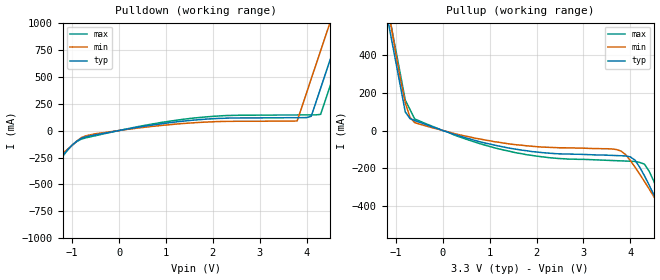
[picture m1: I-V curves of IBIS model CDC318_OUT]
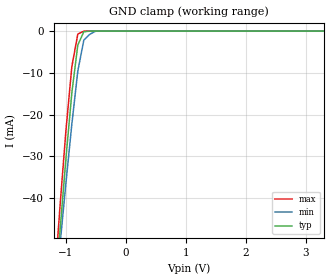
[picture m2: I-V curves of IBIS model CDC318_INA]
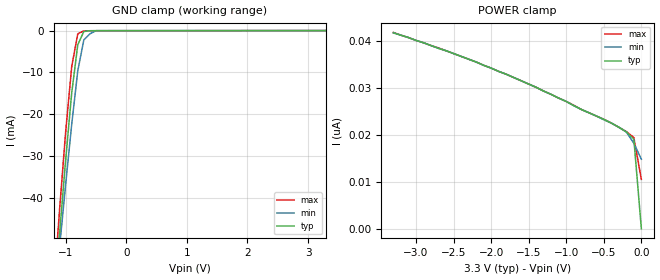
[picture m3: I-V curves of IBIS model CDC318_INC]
[IBIS Ver]   2.1
[File Name]   cd319a10.ibs
[File Rev]   1.0
[Date]   4/15/98
[Source]   file originated at Texas Instruments
[Notes]   The following information corresponds to the
|   CDC319A-DIE output buffers and input ESD circuits, derived
|   from CDC318C, the master chip of CDC319A.
|   Model names kept unchanged to show their equivalent
|   to CDC318C.
|   Only the package paracitics have been changed.
|Revision log: 1.0, 4/15/98  first revision derived from CD318C12.IBS
[Disclaimer] This information is for modeling purposes only
|and is not guaranteed.
|Property of Texas Instruments Incorporated unauthorized reproduction
|and/or distribution is strictly prohibited.
|This product is protected under copyright law and trade
|secret law as an unpublished work.  Created  1997.
|(C) Copyright 1997 Texas Instruments Incorporated.
|All rights reserved.
|These commodities are under U.S. Government distribution
|license control. As such, they are not to be re-exported
|without prior approval of the U.S. Department of Commerce.
|Please be aware that in the absence of a written agreement
|to the contrary, Texas Instruments ("TI") assumes no
|liability for:  (1) the accuracy of the IBIS Models provided
|to your company;  (2) the proper functioning of these Models
|in your design system or for any resulting applications;
|or (3) infringement of patents, copyrights or intellectual
|property rights resulting from your use of these models.
|TI provides IBIS Models as a service to our customers
|and therefore reserves the right to limit distribution
|of the Models.
|CDC319 IBIS I/O Model
|Mixed Signal Products, Texas Instruments
[Component]   CDC319   | 28-pin, DB - package
[Manufacturer] Texas Instruments
[Package]
|   typ   min   max
R_pkg   0.034   0.028   0.039
L_pkg   3.404n   2.704n   4.545n
C_pkg   0.428p   0.299p   0.571p
[Pin]  signal_name   model_name   R_pin   L_pin   C_pin
  1   VCC   POWER   0.038   4.545n   0.564p
  2   1Y0   CDC318_OUT   0.039   4.133n   0.571p
  3   1Y1   CDC318_OUT   0.035   3.598n   0.489p
  4   GND   GND   0.028   3.087n   0.408p
  5   VCC   POWER   0.032   2.990n   0.349p
  6   1Y2   CDC318_OUT   0.032   2.774n   0.318p
  7   1Y3   CDC318_OUT   0.031   2.704n   0.299p
  8   GND   GND   0.031   2.704n   0.299p
  9   A   CDC318_INA   0.032   2.774n   0.318p
 10   VCC   POWER   0.032   2.990n   0.349p
 11   3Y0   CDC318_OUT   0.028   3.087n   0.408p
 12   GND   GND   0.035   3.598n   0.489p
 13   VCC   POWER   0.039   4.133n   0.571p
 14   SDATA   CDC318_IO   0.038   4.545n   0.564p
 15   SCLOCK   CDC318_INC   0.038   4.545n   0.564p
 16   GND   GND   0.039   4.133n   0.571p
 17   GND   GND   0.035   3.597n   0.489p
 18   3Y1   CDC318_OUT   0.028   3.087n   0.408p
 19   VCC   POWER   0.032   2.990n   0.349p
 20   OE   CDC318_INE   0.031   2.774n   0.318p
 21   GND   GND   0.031   2.704n   0.299p
 22   2Y0   CDC318_OUT   0.031   2.704n   0.299p
 23   2Y1   CDC318_OUT   0.032   2.774n   0.318p
 24   VCC   POWER   0.032   2.990n   0.349p
 25   GND   GND   0.028   3.087n   0.408p
 26   2Y2   CDC318_OUT   0.035   3.598n   0.489p
 27   2Y3   CDC318_OUT   0.039   4.133n   0.571p
 28   VCC   POWER   0.038   4.545n   0.564p
| Models and submodels in the file (5): CDC318_OUT (3-state), CDC318_INA (Input), CDC318_INC (Input), CDC318_INE (Input), CDC318_IO (I/O_open_drain)
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|   Model CDC318_OUT
[Model]   CDC318_OUT
Model_type   3-state
Polarity   Non-Inverting
Enable   Active-High
Vmeas = 1.5V
Cref = 30pF
Rref = 500
Vref = 0
|   variable   typ   min   max
C_comp   5.2pF   NA   NA
[Voltage range]   3.3   3.135   3.465
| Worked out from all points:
|   slope of the pulldown table from 0 to 0.495 V, typ, clamps not added: 13.5 ohm
|   slope of the pullup table from 0 to 0.495 V, typ, clamps not added: 12.8 ohm
[Pullup]
| Voltage   I(typ)   I(min)   I(max)
-3.3V     3.358A     3.431A     3.418A
-1.2V     619mA      691mA      682mA
-1.1V     489mA      548mA      551mA
-800mV    98mA       146mA      160mA
-600mV    53mA       42mA       61mA
1.5V      -96mA      -73mA      -114mA
3.8V      -133mA     -108mA     -160mA
4.1V      -156mA     -193mA     -163mA
4.3V      -238mA     -268mA     -177mA
4.9V      -554mA     -514mA     -527mA
5V        -608mA     -556mA     -597mA
6.6V      -1.483A    -1.229A    -1.711A
[Pulldown]
|  Voltage   I(typ)   I(min)   I(max)
-3.3V     -1.354A    -1.086A    -1.669A
-2.6V     -975mA     -790mA     -1.192A
-2.3V     -813mA     -664mA     -989mA
-800mV    -71mA      -65mA      -79mA
1.6V      97mA       72mA       116mA
3.8V      119mA      89mA       144mA
4.1V      132mA      480mA      145mA
4.3V      392mA      740mA      150mA
4.5V      652mA      1A         409mA
4.7V      912mA      1.261A     669mA
4.9V      1.172A     1.521A     929mA
6.6V      3.384A     3.734A     3.137A
[Ramp]
|  variable   typ   min   max
dV/dt_r   2.00/0.95n   2.00/1.05n   2.00/0.85n
dV/dt_f   2.00/1.05n   2.00/1.15n   2.00/0.95n
|   Model CDC318_INA
[Model]   CDC318_INA
Model_type   Input
Polarity   Non-Inverting
Vinl = 0.8V
Vinh = 2.0V
Vmeas = 1.5V
| variable   typ   min   max
C_comp   3.2p   NA   NA
[Voltage range]   3.3   3.135   3.465
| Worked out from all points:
|   GND clamp passes 1 mA (typ) near -0.73 V on its own axis
[GND_Clamp]
|  Voltage   I(typ)   I(min)   I(max)
-3.3V     -477mA     -423mA     -533mA
-1.2V     -66.5mA    -66.7mA    -62.4mA
-1.1V     -48.3mA    -51.6mA    -42.5mA
-1V       -30.8mA    -36.6mA    -24.1mA
-900mV    -14.8mA    -22.3mA    -8.52mA
-800mV    -3.33mA    -9.56mA    -713uA
-700mV    -173uA     -2.17mA    -14.7uA
-600mV    -5.36uA    -765uA     -268nA
-500mV    -161nA     -3.46uA    -6.3nA
3.3V      6.3pA      10nA       10nA
|   Model CDC318_INC
[Model]   CDC318_INC
Model_type   Input
Polarity   Non-Inverting
Vinl = 0.99V
Vinh = 2.31V
Vmeas = 1.5V
| variable   typ   min   max
C_comp   3.2p   NA   NA
[Voltage range]   3.3   3.135   3.465
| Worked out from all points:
|   GND clamp passes 1 mA (typ) near -0.72 V on its own axis
[GND_Clamp]
|  Voltage   I(typ)   I(min)   I(max)
-3.3V     -478mA     -423mA     -534mA
-1.2V     -66.7mA    -66.9mA    -62.6mA
-1.1V     -48.4mA    -51.7mA    -42.7mA
-1V       -30.9mA    -36.7mA    -24.2mA
-900mV    -14.9mA    -22.4mA    -8.6mA
-800mV    -3.39mA    -9.62mA    -777uA
-700mV    -218uA     -2.22mA    -63.8uA
-600mV    -36.4uA    -791uA     -41.6uA
-500mV    -26.1uA    -16.8uA    -39.8uA
3.3V      9.61pA     -20.2nA    -865nA
[POWER_clamp]
|  Voltage   I(typ)   I(min)   I(max)
-3.3V     41.7nA     41.7nA     41.8nA
-2.6V     37.9nA     37.9nA     37.9nA
-1.8V     32.9nA     32.9nA     32.9nA
-1.4V     30.1nA     30.1nA     30.1nA
-1V       27.1nA     27.1nA     27.1nA
-800mV    25.4nA     25.4nA     25.4nA
-500mV    23.3nA     23.2nA     23.3nA
-400mV    22.5nA     22.5nA     22.5nA
-200mV    20.6nA     20.6nA     20.7nA
-100mV    19.1nA     18.2nA     19.4nA
0V        9.61pA     14.8nA     10.5nA
